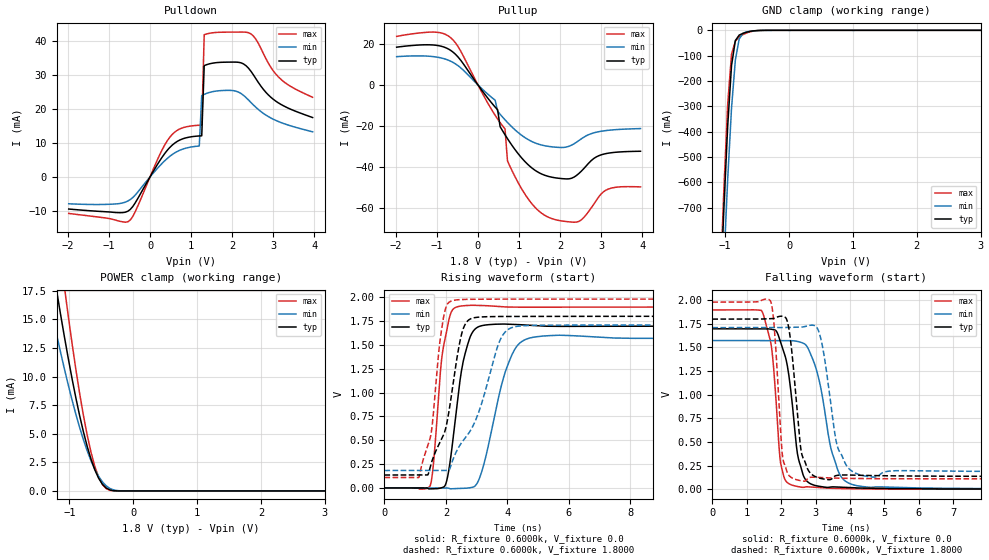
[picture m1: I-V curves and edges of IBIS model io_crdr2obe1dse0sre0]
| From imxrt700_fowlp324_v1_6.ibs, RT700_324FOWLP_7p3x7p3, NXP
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[Model] io_crdr2obe1dse0sre0
|   Model io_crdr2obe1dse0sre0
| This model was characterised for following simulation conditions:
| External (pad) voltage:
|   - Typ: 1.8V,   - Min: 1.71V,   - Max: 1.98V
| Library cells for typ/min/max conditions are connected as defined below:
|  PAD_IO - External Pad
|  ipp_do - Core Input
|  ipp_obe - Output Buffer Enable
|  ASRCN3V3[3] - NC
|  ASRCN3V3[4] - NC
|  ASRCP3V3[4] - NC
|  REFAPBIAS3V3 - gnde
|  REFBAMPL3V3 - vdd1v8
|  REFCAMPH3V3 - vdd1v8
|  REFDNBIAS3V3 - vdd1v8
|  REFH3V3 - REFH3V3
|  REFL3V3 - REFL3V3
|  gnde - gnde
|  ipp_dse - gnde
|  ipp_ina235_3v - NC
|  ipp_ina40_3v - NC
|  ipp_ina_mux - NC
|  ipp_ind - NC
|  ipp_ind_1p8v - NC
|  ipp_ind_3v - NC
|  ipp_sre - gnde
|  vdd - vdd
|  vdd1v8 - vdd1v8
|  vdda - vdde3v3
|  vdde3v3 - vdde3v3
| All other pins connected to ground
Model_type I/O
Polarity   Non-Inverting
Enable   Active-High
Vinl =   0.5400V
Vinh =   1.2600V
Vmeas =  0.9000V
Cref =   15.0000pF
Rref =   0.6000k
Vref =   0.0V
C_comp   3.9792pF   3.7942pF   4.1043pF
|C_comp_pullup   0.4867pF   0.5823pF   0.4754pF
|C_comp_pulldown   2.0824pF   2.1676pF   1.8520pF
[Model Spec]
| variable   typ   min   max
Vinh   1.2600V   NA   NA
Vinl   0.5400V   NA   NA
Vref   0.0V   0.0V   0.0V
Cref   15.0000pF   15.0000pF   15.0000pF
Rref   0.6000k   0.6000k   0.6000k
[Receiver Thresholds]
Vcross_high  =   0.0V
Vcross_low  =   0.0V
Vdiff_ac  =   0.0V
Vdiff_dc  =   0.0V
Tdiffslew_ac  =   0.0S
[Temperature Range]   25.0000   0.1250k   -40.0000
[Voltage Range]   1.8000V   1.7100V   1.9800V
[Pullup Reference]   1.8000V   1.7100V   1.9800V
[Pulldown Reference]   0.0V   0.0V   0.0V
[POWER Clamp Reference]   1.8000V   1.7100V   1.9800V
[GND Clamp Reference]   0.0V   0.0V   0.0V
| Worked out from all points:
|   slope of the pulldown table from 0 to 0.27 V, typ, clamps not added: 50.4 ohm
|   slope of the pullup table from 0 to 0.27 V, typ, clamps not added: 37.4 ohm
|   GND clamp passes 1 mA (typ) near -0.50 V on its own axis
|   POWER clamp passes 1 mA (typ) near -0.53 V on its own axis
|   rising waveform, R_fixture 0.6000k, V_fixture 0.0: 20-80 % time 421ps typ, 689ps min, 313ps max; typ from 0 V to 1.7 V
|   rising waveform, R_fixture 0.6000k, V_fixture 1.8000: 20-80 % time 623ps typ, 1.07ns min, 382ps max; typ from 0.135 V to 1.8 V
|   falling waveform, R_fixture 0.6000k, V_fixture 0.0: 20-80 % time 340ps typ, 519ps min, 239ps max; typ from 1.7 V to 0 V
|   falling waveform, R_fixture 0.6000k, V_fixture 1.8000: 20-80 % time 249ps typ, 358ps min, 184ps max; typ from 1.8 V to 0.135 V
[Pulldown]
|Voltage   I(typ)   I(min)   I(max)
-1.98V    -9.436mA   -7.894mA   -10.73mA
-480mV    -9.54mA    -6.639mA   -12.65mA
480mV     8.647mA    6.046mA    11.65mA
780mV     11.13mA    8.114mA    14.39mA
1.2V      12.06mA    9.104mA    15.21mA
1.26V     12.11mA    23.94mA    15.24mA
1.32V     32.75mA    24.29mA    41.84mA
2.04V     33.78mA    25.37mA    42.6mA
2.46V     31.05mA    21.88mA    42.06mA
2.82V     24.92mA    18.21mA    34.86mA
3.12V     21.84mA    16.34mA    29.51mA
3.96V     17.47mA    13.28mA    23.42mA
[Pullup]
|Voltage   I(typ)   I(min)   I(max)
-1.98V    18.38mA    13.75mA    23.61mA
-600mV    15.86mA    10.88mA    21.76mA
420mV     -10.83mA   -7.487mA   -14.84mA
480mV     -12.18mA   -12.88mA   -16.66mA
540mV     -20.35mA   -14.31mA   -18.38mA
660mV     -24.32mA   -17.04mA   -21.51mA
720mV     -26.22mA   -18.33mA   -37.1mA
900mV     -31.46mA   -21.85mA   -44.64mA
1.62V     -44.01mA   -29.64mA   -63.5mA
2.4V      -44.17mA   -27.97mA   -66.91mA
3.12V     -33.49mA   -22.27mA   -51.3mA
3.96V     -32.36mA   -21.31mA   -49.74mA
[GND_clamp]
|Voltage   I(typ)   I(min)   I(max)
-1.98V    -7.543A    -7.6A      -7.897A
-1.08V    -1.077A    -1.286A    -1.025A
-1.02V    -705.3mA   -921.3mA   -628.8mA
-960mV    -377.1mA   -587.4mA   -291.7mA
-900mV    -139.2mA   -307mA     -94.38mA
-840mV    -40.12mA   -117mA     -42.82mA
-780mV    -18.81mA   -33.95mA   -26.13mA
-720mV    -11.86mA   -11.44mA   -16.78mA
-660mV    -7.061mA   -5.737mA   -9.992mA
-540mV    -1.684mA   -1.901mA   -2.15mA
-420mV    -207.1uA   -403.7uA   -160.6uA
3.96V     0A         0A         0A
[POWER_clamp]
|Voltage   I(typ)   I(min)   I(max)
-1.98V    46.79mA    35.94mA    61.38mA
-1.32V    21.77mA    16.85mA    28.91mA
-1.2V     17.57mA    13.71mA    23.33mA
-1.14V    15.55mA    12.2mA     20.62mA
-1.08V    13.59mA    10.75mA    17.99mA
-1.02V    11.7mA     9.353mA    15.46mA
-900mV    8.209mA    6.76mA     10.73mA
-720mV    3.898mA    3.51mA     4.887mA
-540mV    1.103mA    1.267mA    1.195mA
-420mV    244.5uA    429.2uA    190.6uA
-180mV    280.9nA    5.273uA    26.8nA
3.96V     0A         0A         0A
[Ramp]
| variable   typ   min   max
dV/dt_r  1.0186/0.4209n   0.9439/0.6893n   1.1383/0.3129n
dV/dt_f  0.9990/0.2490n   0.9166/0.3581n   1.1224/0.1844n
R_load = 0.6000k
[Rising Waveform]
R_fixture= 0.6000k
V_fixture= 0.0
V_fixture_min= 0.0
V_fixture_max= 0.0
|time   V(typ)   V(min)   V(max)
0s        115.1nV    3.181uV    43.69nV
1.485ns   -10.23mV   -972.1uV   19.71mV
1.591ns   -8.91mV    -1.171mV   237.6mV
1.921ns   8.672mV    -862.3uV   1.482V
2.183ns   382.6mV    -8.946mV   1.849V
2.56ns    1.32V      -5.192mV   1.909V
3.103ns   1.695V     109.2mV    1.913V
4.237ns   1.714V     1.451V     1.895V
5.144ns   1.697V     1.592V     1.895V
60ns      1.698V     1.573V     1.897V
[Rising Waveform]
R_fixture= 0.6000k
V_fixture= 1.8000
V_fixture_min= 1.7100
V_fixture_max= 1.9800
|time   V(typ)   V(min)   V(max)
0s        135mV      182.4mV    109.3mV
1.122ns   134.2mV    182.3mV    111.7mV
1.52ns    255.1mV    181.5mV    571.9mV
1.778ns   458.4mV    181.8mV    1.46V
1.954ns   580.4mV    182.4mV    1.837V
2.365ns   1.373V     396.1mV    1.972V
2.767ns   1.766V     584.4mV    1.978V
3.796ns   1.798V     1.571V     1.979V
4.517ns   1.798V     1.7V       1.979V
60ns      1.8V       1.71V      1.98V
[Falling Waveform]
R_fixture= 0.6000k
V_fixture= 0.0
V_fixture_min= 0.0
V_fixture_max= 0.0
|time   V(typ)   V(min)   V(max)
0s        1.698V     1.573V     1.897V
1.441ns   1.699V     1.573V     1.883V
1.716ns   1.693V     1.573V     1.51V
1.873ns   1.665V     1.573V     819.6mV
2.092ns   1.435V     1.574V     117.7mV
2.632ns   156.2mV    1.546V     18.48mV
3.041ns   34.44mV    1.245V     17.23mV
3.684ns   21.52mV    168.7mV    6.833mV
4.563ns   9.707mV    19.96mV    2.319mV
60ns      6.619uV    14.16uV    1.062uV
[Falling Waveform]
R_fixture= 0.6000k
V_fixture= 1.8000
V_fixture_min= 1.7100
V_fixture_max= 1.9800
|time   V(typ)   V(min)   V(max)
0s        1.8V       1.71V      1.98V
1.691ns   1.804V     1.71V      1.991V
1.819ns   1.813V     1.709V     1.623V
2.06ns    1.829V     1.71V      303mV
2.252ns   1.635V     1.712V     135.5mV
2.645ns   322.9mV    1.718V     84.87mV
3.125ns   115.6mV    1.632V     123.6mV
3.672ns   148.2mV    413.6mV    116.2mV
4.643ns   144.1mV    128.1mV    111.4mV
60ns      135mV      182.4mV    109.3mV
